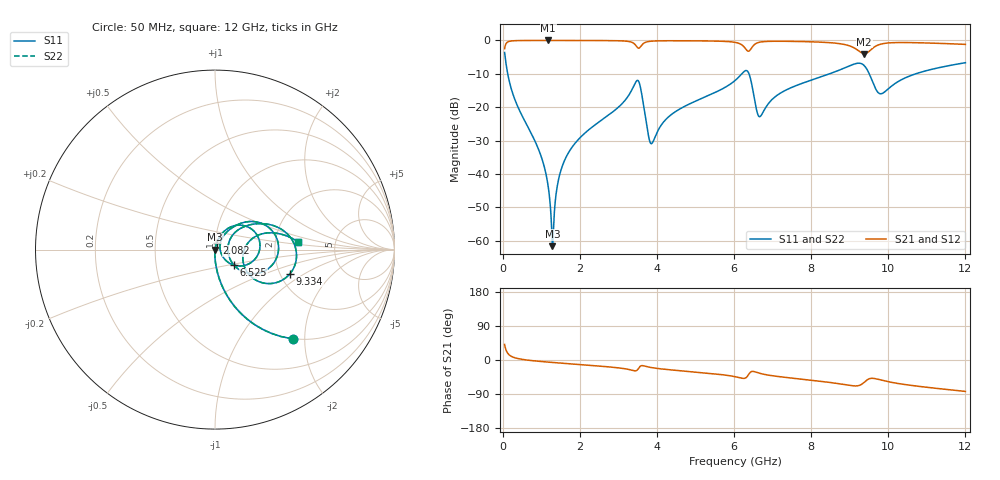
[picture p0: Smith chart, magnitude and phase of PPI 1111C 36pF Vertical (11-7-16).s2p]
# GHz S MA R 50
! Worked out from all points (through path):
!   1601 points, 50 MHz to 12 GHz, reference 50 ohm
!   highest |S21| = -0.01 dB at 1.178 GHz (marker M1); lowest = -4.0 dB at 9.378 GHz (marker M2)
!   group delay of S21, straight-line fit = 19 ps
!   lowest |S11| = -61.6 dB at 1.29 GHz (marker M3), VSWR 1.00, Z = 50.1 - j0.0269 ohm
!   |S11| at or under -10 dB: 130.7 MHz to 6.201 GHz (6.071 GHz wide, 192 % of centre); 6.388 GHz to 8.476 GHz (2.088 GHz wide, 28.1 % of centre); 9.506 GHz to 10.71 GHz (1.206 GHz wide, 11.9 % of centre)
!   |S22| runs from -61.6 to -3.6 dB; largest |S21 - S12| = 0
!   S11 on the Smith chart (normalised r, x): 50 MHz: 0.99, -1.75; 2.082 GHz: 1.02, +0.08; 6.525 GHz: 1.22, -0.22; 9.334 GHz: 2.27, -0.75; 12 GHz: 2.69, +0.31
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0.05  0.6601 -48.9  0.751 41.1  0.751 41.1  0.6601 -48.9
0.2441875  0.1714 -81.2  0.9848 8.6  0.9848 8.6  0.1714 -81.2
0.9537187  0.02155 -91.7  0.999 -3.6  0.999 -3.6  0.02155 -91.7
1.177781  0.006647 -88.9  0.9991 -5.6  0.9991 -5.6  0.006647 -88.9
1.289813  0.0008283 -18.9  0.9991 -6.5  0.9991 -6.5  0.0008283 -18.9
1.536281  0.01262 77.5  0.9989 -8.5  0.9989 -8.5  0.01262 77.5
2.044156  0.0367 75.8  0.998 -12.4  0.998 -12.4  0.0367 75.8
2.0815  0.03849 75.5  0.9979 -12.7  0.9979 -12.7  0.03849 75.5
3.485625  0.2514 14.0  0.796 -26.9  0.796 -26.9  0.2514 14.0
3.821719  0.02999 -9.7  0.9702 -19.3  0.9702 -19.3  0.02999 -9.7
4.038312  0.0459 50.4  0.9854 -22.6  0.9854 -22.6  0.0459 50.4
6.025  0.2507 38.7  0.9361 -44.0  0.9361 -44.0  0.2507 38.7
6.338687  0.3509 -4.2  0.7044 -44.0  0.7044 -44.0  0.3509 -4.2
6.525406  0.1369 -39.3  0.8641 -30.7  0.8641 -30.7  0.1369 -39.3
6.68225  0.07291 8.1  0.9455 -35.5  0.9455 -35.5  0.07291 8.1
8.019156  0.2563 33.6  0.9532 -53.5  0.9532 -53.5  0.2563 33.6
8.900469  0.3944 15.7  0.86 -65.5  0.86 -65.5  0.3944 15.7
9.333656  0.4395 -17.7  0.6383 -62.4  0.6383 -62.4  0.4395 -17.7
9.378469  0.4183 -23.1  0.6291 -58.7  0.6291 -58.7  0.4183 -23.1
9.744438  0.164 -18.8  0.857 -51.1  0.857 -51.1  0.164 -18.8
10.01331  0.1912 12.4  0.9177 -57.6  0.9177 -57.6  0.1912 12.4
12  0.464 5.5  0.8729 -82.9  0.8729 -82.9  0.464 5.5
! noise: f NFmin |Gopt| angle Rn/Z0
0.05  0.0003363  0.8535  0.8888  0.0004899
1.372  0.003342  0.6412  6.891  0.001754
2.701  0.008121  0.7012  13.28  0.005255
4.031  0.02256  0.8298  20.03  0.02708
5.36  0.01831  0.7399  26.05  0.0134
6.682  0.057  0.8894  32.6  0.1033
8.012  0.03052  0.7741  38.11  0.0247
9.341  0.1956  0.956  44.38  0.8584
10.67  0.04753  0.8146  49.56  0.04424
12  0.03649  0.7486  54  0.02332
